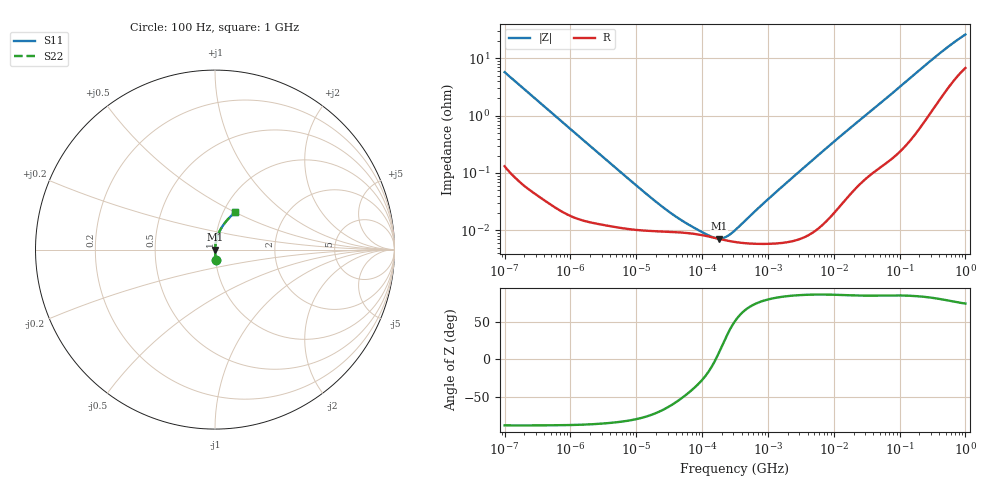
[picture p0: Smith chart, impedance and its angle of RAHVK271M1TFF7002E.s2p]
! RAHVK271M1TFF7002E  S-PARAMETER MODEL  (AEC-Q200 qualified)
! Model Generated by ELNA Corporation (http://www.ty-top.com)
! Version 1.0
! ELNA Control No. 201216
! Copyright (c) 2020 ELNA CO.,LTD. All Rights Reserved.
! Products Name : CONDUCTIVE POLYMER HYBRID ALUMINUM ELECTROLYTIC CAPACITORS
! Characteristics :
!  Capacitance  :  270uF  ,  Rated voltage  :  25V
!  Operating Temp. Range  :  -55 to +125 degC  ,  Endurance  :  4000hr at 125 degC
!  Dimension D  :  10mm  ,  Dimension L  :  8.7mm
! Frequency Range : 100Hz - 1GHz
! External Node Assignments :
!  1  o---| |---o  2
# MHz S RI R 50
!Freq[MHz].  S11 Real  S11 Imag  S21 Real  S21 Imag  S12 Real  S12 Imag  S22 Real  S22 Imag
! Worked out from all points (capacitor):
!   401 points, 100 Hz to 1 GHz, reference 50 ohm
!   read as one part in series: C = 276 uF near 108 Hz
!   lowest |Z| = 7.2 mohm at 179.9 kHz (marker M1)
!   series resonance near 161.1 kHz, so ESL is about 3.5 nH
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0.0001  0.0046 -0.0572  0.9954 0.0572  0.9954 0.0572  0.0046 -0.0572
0.000113  0.0037 -0.0508  0.9963 0.0508  0.9963 0.0508  0.0037 -0.0508
0.000309  0.000762 -0.0187  0.9992 0.0187  0.9992 0.0187  0.000762 -0.0187
0.001488  0.000166 -0.00395  0.9998 0.00395  0.9998 0.00395  0.000166 -0.00395
0.009495  0.000103 -0.000631  0.9999 0.000631  0.9999 0.000631  0.000103 -0.000631
0.022131  9.6e-05 -0.00027  0.9999 0.00027  0.9999 0.00027  9.6e-05 -0.00027
0.04217  9.27e-05 -0.000139  0.9999 0.000139  0.9999 0.000139  9.27e-05 -0.000139
0.083657  8.54e-05 -5.97e-05  0.9999 5.97e-05  0.9999 5.97e-05  8.54e-05 -5.97e-05
0.098288  8.28e-05 -4.5e-05  0.9999 4.5e-05  0.9999 4.5e-05  8.28e-05 -4.5e-05
0.179887  7.12e-05 1.1e-05  0.9999 -1.1e-05  0.9999 -1.1e-05  7.12e-05 1.1e-05
0.291743  6.36e-05 6.71e-05  0.9999 -6.71e-05  0.9999 -6.71e-05  6.36e-05 6.71e-05
0.316228  6.27e-05 7.81e-05  0.9999 -7.81e-05  0.9999 -7.81e-05  6.27e-05 7.81e-05
0.342768  6.18e-05 8.98e-05  0.9999 -8.98e-05  0.9999 -8.98e-05  6.18e-05 8.98e-05
1.102808  5.85e-05 0.00038  0.9999 -0.00038  0.9999 -0.00038  5.85e-05 0.00038
4.704354  9.28e-05 0.00166  0.9999 -0.00166  0.9999 -0.00166  9.28e-05 0.00166
14.53784  0.00035 0.00502  0.9996 -0.00502  0.9996 -0.00502  0.00035 0.00502
69.9842  0.00213 0.0222  0.9979 -0.0222  0.9979 -0.0222  0.00213 0.0222
176.8072  0.00785 0.0543  0.9921 -0.0543  0.9921 -0.0543  0.00785 0.0543
395.8221  0.0309 0.1124  0.9691 -0.1124  0.9691 -0.1124  0.0309 0.1124
668.3439  0.069 0.1658  0.931 -0.1658  0.931 -0.1658  0.069 0.1658
922.5714  0.1036 0.2009  0.8964 -0.2009  0.8964 -0.2009  0.1036 0.2009
1000  0.1133 0.2098  0.8867 -0.2098  0.8867 -0.2098  0.1133 0.2098
